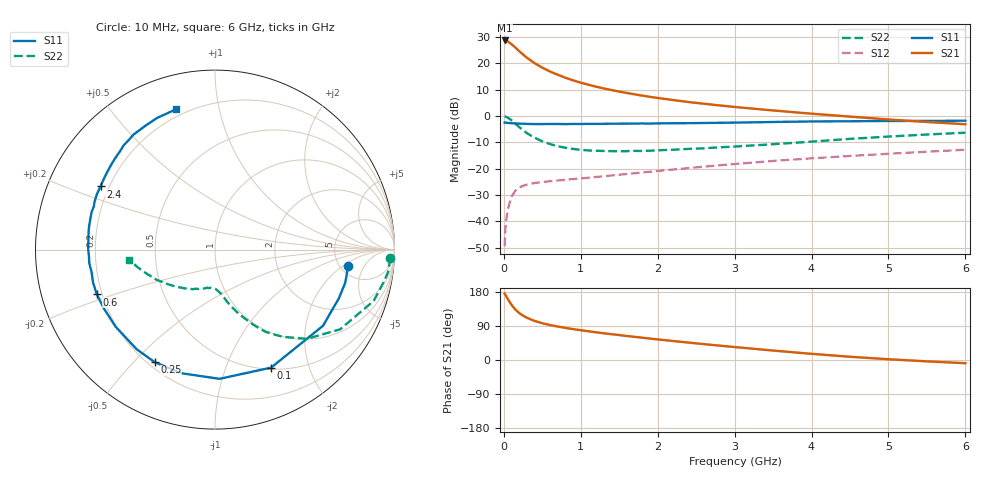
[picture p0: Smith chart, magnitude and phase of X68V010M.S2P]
! SIEMENS Small Signal Semiconductors
! BFP193W
! Si NPN RF Bipolar Junction Transistor in SOT343
! VCE = 8 V  IC = 10 mA
! Common Emitter S-Parameters:  April 1994
# GHz  S  MA  R  50
!  f  S11  S21  S12  S22
! GHz  MAG  ANG  MAG  ANG  MAG  ANG  MAG  ANG
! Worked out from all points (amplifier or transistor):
!   40 points, 10 MHz to 6 GHz, reference 50 ohm
!   highest |S21| = 28.6 dB at 10 MHz (marker M1)
!   |S21| within 3 dB of that: start of sweep to 161.2 MHz
!   unconditionally stable (mu >= 1): 1.38 GHz to 4.535 GHz
!   at 200 MHz: K = 0.21, MSG = 25.9 dB, |S12| = -27.2 dB
!   at 1.5 GHz: K = 1.04, MAG = 14.6 dB, |S12| = -22.3 dB
!   at 6 GHz: K = 0.92, MSG = 4.8 dB, |S12| = -12.8 dB
!   lowest NFmin = 1.30 dB at 450 MHz
!   S11 on the Smith chart (normalised r, x): 10 MHz: 5.92, -2.41; 100 MHz: 0.52, -1.45; 250 MHz: 0.23, -0.58; 600 MHz: 0.18, -0.18; 2.4 GHz: 0.17, +0.25; 6 GHz: 0.16, +0.75
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0.01  0.7478 -6.9  26.92 175.1  0.0034 87.8  0.978 -2.8
0.02  0.7488 -14.2  26.87 172.2  0.0072 81.1  0.9719 -7.5
0.03  0.7417 -21.4  26.62 168.6  0.0103 80.3  0.9572 -10.9
0.05  0.7364 -35.2  25.85 161.3  0.0167 74.4  0.9291 -17.9
0.1  0.7281 -64.6  22.94 145.6  0.0296 60.0  0.8268 -32.5
0.15  0.7204 -88.0  19.75 133.0  0.0383 50.5  0.7132 -44.2
0.2  0.714 -105.3  16.85 123.8  0.0437 44.2  0.6139 -52.3
0.25  0.7114 -118.1  14.56 116.9  0.0474 39.4  0.537 -58.5
0.3  0.7063 -128.1  12.65 111.4  0.0499 36.7  0.4711 -62.9
0.4  0.7008 -142.1  9.991 103.1  0.0535 33.1  0.3856 -69.4
0.5  0.7007 -152.1  8.211 97.0  0.0559 31.9  0.3299 -74.0
0.6  0.7041 -159.2  6.937 92.2  0.0578 31.6  0.2926 -77.4
0.8  0.6989 -169.7  5.29 84.7  0.0614 32.5  0.2495 -82.1
1.1  0.7068 179.8  3.904 75.8  0.0674 35.5  0.2214 -88.3
1.3  0.7088 174.2  3.314 70.5  0.0719 37.5  0.2164 -92.0
1.6  0.7146 167.2  2.723 63.3  0.0793 40.2  0.215 -97.3
2.2  0.7269 154.9  2 50.1  0.0963 43.7  0.2284 -108.6
2.4  0.7284 151.1  1.835 46.0  0.1026 44.2  0.2371 -112.1
3.2  0.7544 137.4  1.391 30.5  0.1292 44.4  0.2738 -127.8
4.5  0.792 119.1  0.97 8.5  0.1741 40.3  0.3673 -152.9
5.5  0.8039 109.9  0.767 -3.6  0.2098 35.7  0.4442 -167.5
6  0.8116 105.5  0.696 -8.5  0.2287 33.5  0.4805 -173.3
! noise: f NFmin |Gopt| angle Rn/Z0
0.45  1.3  0.22  143  0.11
0.9  1.3  0.34  160  0.11
1.8  2.05  0.54  -153  0.14
